PROGRAM p02_SFC
VAR
	M0: BOOL;
	M1: BOOL;
	S0: BOOL;
	S1: BOOL;
END_VAR

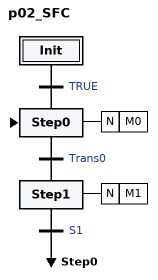
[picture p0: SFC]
INITIAL_STEP Init:
END_STEP
TRANSITION FROM Init TO Step0
    := TRUE;
END_TRANSITION
STEP Step0:
    M0(N);
END_STEP
TRANSITION FROM Step0 TO Step1
    := Trans0;
END_TRANSITION
STEP Step1:
    M1(N);
END_STEP
TRANSITION FROM Step1 TO Step0
    := S1;
END_TRANSITION

TRANSITION Trans0:
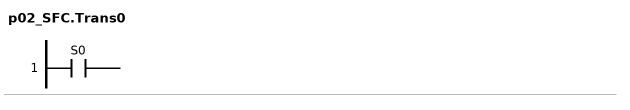
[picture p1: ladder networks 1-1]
// NETWORK 1
(* S0; not connected *)
END_TRANSITION

END_PROGRAM
